[IBIS VER]   5.0
[File Name]   am13e230pn.ibs
[File Rev]   1.0
[Date]   February 08, 2026
[Source]   File originated at Texas Instruments
[Copyright]   (c) 2012, Texas Instruments Inc.
[Component]   am13e230pn
[Manufacturer] Texas Instruments
[Package]
| Variable   Typ   Min   Max
   R_pkg 2.94E-01 1.43E-01 3.97E-01
   L_pkg 6.08E-09 4.47E-09 7.53E-09
   C_pkg 1.84E-14 1.43E-14 3.70E-14
[Pin]   signal_name   model_name   R_pin   L_pin   C_pin
   1   VDD   NC 3.05E-01 6.58E-09 3.04E-14
   2   PB13   BCF3385DSWHYPBFZSD_87U 2.86E-01 6.29E-09 1.79E-14
   3   PB14   BCF3385DSHYPBFZSD_87U 2.74E-01 6.08E-09 1.74E-14
   4   PB15   BCF3385DSHYPBFZSD_87U 2.65E-01 5.90E-09 1.69E-14
   5 PC16_X1   BCF3385DSHYPBFZSD_87U 2.78E-01 5.95E-09 1.66E-14
   6 PC17_X2   BCF3385DSHYPBFZSD_87U 2.78E-01 5.86E-09 1.62E-14
   7   NRST   BQ0491FSSD_XRSN_87U 2.72E-01 5.71E-09 1.57E-14
   8   PB0   BCF3385DSHYPBFZSD_87U 2.65E-01 5.55E-09 1.53E-14
   9   PB1   BCF3385DSWHYPBFZSD_87U 2.61E-01 5.42E-09 1.48E-14
   10   PB2   BCF3385DSHYPBFZSD_87U 2.60E-01 5.32E-09 1.44E-14
   11   PB3   BCF3385DSHYPBFZSD_87U 2.60E-01 5.32E-09 1.44E-14
   12   PA0   BCF3385DSWHYPBFZSD_87U 2.59E-01 5.40E-09 1.48E-14
   13   PA1   BCF3385DSHYPBFZSD_87U 2.57E-01 5.47E-09 1.52E-14
   14   PA2   BCF3385DSWHYPBFZSD_87U 2.58E-01 5.56E-09 1.56E-14
   15   VSSA   NC 1.43E-01 4.47E-09 1.80E-14
   16   VDDA   NC 1.45E-01 4.57E-09 1.84E-14
   17   PA3   BCF3385DSHYPBFZSD_87U 2.71E-01 5.96E-09 1.70E-14
   18   PA4   BCF3385DSHYPBFZSD_87U 3.06E-01 6.41E-09 1.76E-14
   19   PA5   BCF3385DSHYPBFZSD_87U 3.26E-01 6.71E-09 1.82E-14
   20   PA6   BCF3385DSHYPBFZSD_87U 3.50E-01 7.04E-09 3.11E-14
   21   PA7   BCF3385DSHYPBFZSD_87U 3.54E-01 7.09E-09 3.12E-14
   22   PB4   BCF3385DSHYPBFZSD_87U 3.40E-01 6.85E-09 1.83E-14
   23   PB5   BCF3385DSWHYPBFZSD_87U 3.28E-01 6.64E-09 1.78E-14
   24   PA16   BCF3385DSHYPBFZSD_87U 3.19E-01 6.47E-09 1.73E-14
   25   PA17   BCF3385DSHYPBFZSD_87U 3.13E-01 6.31E-09 1.69E-14
   26   PA18   BCF3385DSHYPBFZSD_87U 3.09E-01 6.18E-09 1.64E-14
   27   VREFLO   NC 3.09E-01 6.09E-09 1.60E-14
   28   VREFHI   NC 3.09E-01 6.01E-09 1.56E-14
   29   VDDA   NC 3.14E-01 5.97E-09 1.52E-14
   30   PC7   BCF3385DSHYPBFZSD_87U 3.13E-01 5.87E-09 1.48E-14
   31   PC8   BCF3385DSHYPBFZSD_87U 3.10E-01 5.84E-09 1.48E-14
   32   PC9   BCF3385DSHYPBFZSD_87U 3.08E-01 5.91E-09 1.52E-14
   33   PC10   BCF3385DSHYPBFZSD_87U 3.09E-01 6.00E-09 1.56E-14
   34   PC11   BCF3385DSHYPBFZSD_87U 3.12E-01 6.12E-09 1.60E-14
   35   PC12   BCF3385DSHYPBFZSD_87U 3.17E-01 6.26E-09 1.65E-14
   36   PC13   BCF3385DSHYPBFZSD_87U 3.24E-01 6.43E-09 1.70E-14
   37   PC14   BCF3385DSHYPBFZSD_87U 3.34E-01 6.62E-09 1.75E-14
   38   PC15   BCF3385DSHYPBFZSD_87U 3.47E-01 6.84E-09 1.80E-14
   39   PA26   BCF3385DSHYPBFZSD_87U 3.62E-01 7.08E-09 1.85E-14
   40   VSS   NC 2.02E-01 5.52E-09 3.70E-14
   41   VDD   NC 3.75E-01 7.30E-09 3.15E-14
   42   PA27   BCF3385DSHYPBFZSD_87U 3.50E-01 6.95E-09 1.84E-14
   43   PA28   BCF3385DSHYPBFZSD_87U 3.38E-01 6.75E-09 1.79E-14
   44   PA29   BCF3385DSHYPBFZSD_87U 3.30E-01 6.57E-09 1.74E-14
   45   PA30   BCF3385DSHYPBFZSD_87U 3.24E-01 6.42E-09 1.69E-14
   46   PA31   BCF3385DSHYPBFZSD_87U 3.20E-01 6.29E-09 1.65E-14
   47   PB24   BCF3385DSHYPBFZSD_87U 3.18E-01 6.18E-09 1.61E-14
   48   PB25   BCF3385DSHYPBFZSD_87U 3.17E-01 6.09E-09 1.57E-14
   49   PB26   BCF3385DSHYPBFZSD_87U 3.18E-01 6.01E-09 1.53E-14
   50   VSS   NC 3.25E-01 5.99E-09 1.49E-14
   51   VDD   NC 3.25E-01 5.99E-09 1.49E-14
   52   PB6   BCF3385DSHYPBFZSD_87U 3.21E-01 6.04E-09 1.53E-14
   53   PB7   BCF3385DSHYPBFZSD_87U 3.24E-01 6.16E-09 1.57E-14
   54   PB8   BCF3385DSHYPBFZSD_87U 3.22E-01 6.22E-09 1.61E-14
   55   PB9   BCF3385DSHYPBFZSD_87U 3.26E-01 6.36E-09 1.66E-14
   56   PA8   BCF3385DSHYPBFZSD_87U 3.33E-01 6.52E-09 1.70E-14
   57   PA9   BCF3385DSHYPBFZSD_87U 3.43E-01 6.70E-09 1.75E-14
   58   PA10   BCF3385DSHYPBFZSD_87U 3.54E-01 6.91E-09 1.80E-14
   59   PA11   BCF3385DSHYPBFZSD_87U 3.52E-01 6.97E-09 1.84E-14
   60   PA12  BCPF335585DSHYPBFZSD_87U 3.67E-01 7.21E-09 3.13E-14
   61   VSS   NC 3.64E-01 7.19E-09 3.13E-14
   62   VDD   NC 1.80E-01 5.20E-09 2.07E-14
   63   PA13 BCF3385DSHYPBFZSD_TMS_87U 3.11E-01 6.47E-09 1.77E-14
   64   PA14 BCF3385DSHYPBFZSD_TMS_87U 2.63E-01 5.89E-09 1.69E-14
   65   PA15  BCPF335585DSHYPBFZSD_87U 2.55E-01 5.71E-09 1.64E-14
   66   PB10   BCF3385DSHYPBFZSD_87U 2.49E-01 5.57E-09 1.60E-14
   67   PB11   BCF3385DSHYPBFZSD_87U 2.47E-01 5.46E-09 1.56E-14
   68   PB12   BCF3385DSHYPBFZSD_87U 2.47E-01 5.37E-09 1.51E-14
   69   PB16   BCF3385DSHYPBFZSD_87U 2.48E-01 5.29E-09 1.47E-14
   70   PB17   BCF3385DSHYPBFZSD_87U 2.50E-01 5.23E-09 1.43E-14
   71   PB18  BCPF335585DSHYPBFZSD_87U 2.52E-01 5.24E-09 1.43E-14
   72   PA19  BCPF335585DSHYPBFZSD_87U 2.49E-01 5.30E-09 1.47E-14
   73   PA20   BCF3385DSHYPBFZSD_87U 2.51E-01 5.40E-09 1.52E-14
   74   PA21   BCF3385DSHYPBFZSD_87U 2.52E-01 5.50E-09 1.56E-14
   75   PA22   BCF3385DSHYPBFZSD_87U 2.57E-01 5.65E-09 1.60E-14
   76   PA23   BCF3385DSHYPBFZSD_87U 2.66E-01 5.82E-09 1.65E-14
   77   PA24   BCF3385DSHYPBFZSD_87U 2.74E-01 5.99E-09 1.70E-14
   78   PA25   BCF3385DSHYPBFZSD_87U 2.87E-01 6.22E-09 1.75E-14
   79   VSS   NC 1.64E-01 5.04E-09 2.02E-14
   80   VDD   NC 3.01E-01 6.54E-09 3.04E-14
| End of package information
|   Component BCF3385DSHYPBFZSD_87U
[Component] BCF3385DSHYPBFZSD_87U
[Manufacturer] Texas Instruments
[Package]
| variable   typ   min   max
R_pkg   0.0   0.0   0.0
L_pkg   0.0H   0.0H   0.0H
C_pkg   0.0F   0.0F   0.0F
[Pin]  signal_name   model_name   R_pin   L_pin   C_pin
PAD   PAD   BCF3385DSHYPBFZSD_87U
VDDS   VDDS   Power
VSS   VSS   Gnd
A   A   NC
GZ   GZ   NC
[Model Selector] BCF3385DSHYPBFZSD_87U
BCF3385DSHYPBFZSD_87U_PUPDOFF PI=1 PSEL=1
BCF3385DSHYPBFZSD_87U_PDON PI=0 PSEL=0
BCF3385DSHYPBFZSD_87U_PUON PI=0 PSEL=1
|   Component BCF3385DSHYPBFZSD_TMS_87U
[Component] BCF3385DSHYPBFZSD_TMS_87U
[Manufacturer] Texas Instruments
[Package]
| variable   typ   min   max
R_pkg   0.0   0.0   0.0
L_pkg   0.0H   0.0H   0.0H
C_pkg   0.0F   0.0F   0.0F
[Pin]  signal_name   model_name   R_pin   L_pin   C_pin
PAD   PAD   BCF3385DSHYPBFZSD_TMS_87U
VDDS   VDDS   Power
VSS   VSS   Gnd
A   A   NC
GZ   GZ   NC
[Model Selector] BCF3385DSHYPBFZSD_TMS_87U
BCF3385DSHYPBFZSD_TMS_87U_PUPDOFF PI=1 PSEL=1
BCF3385DSHYPBFZSD_TMS_87U_PDON PI=0 PSEL=0
BCF3385DSHYPBFZSD_TMS_87U_PUON PI=0 PSEL=1
|   Component BCF3385DSWHYPBFZSD_87U
[Component] BCF3385DSWHYPBFZSD_87U
[Manufacturer] Texas Instruments
[Package]
| variable   typ   min   max
R_pkg   0.0   0.0   0.0
L_pkg   0.0H   0.0H   0.0H
C_pkg   0.0F   0.0F   0.0F
[Pin]  signal_name   model_name   R_pin   L_pin   C_pin
PAD   PAD   BCF3385DSWHYPBFZSD_87U
VDDS   VDDS   Power
VSS   VSS   Gnd
A   A   NC
GZ   GZ   NC
[Model Selector] BCF3385DSWHYPBFZSD_87U
BCF3385DSWHYPBFZSD_87U_PUPDOFF PI=1 PSEL=1
BCF3385DSWHYPBFZSD_87U_PDON PI=0 PSEL=0
BCF3385DSWHYPBFZSD_87U_PUON PI=0 PSEL=1
|   Component BCPF335585DSHYPBFZSD_87U
[Component] BCPF335585DSHYPBFZSD_87U
[Manufacturer] Texas Instruments
[Package]
| variable   typ   min   max
R_pkg   0.0   0.0   0.0
L_pkg   0.0H   0.0H   0.0H
C_pkg   0.0F   0.0F   0.0F
[Pin]  signal_name   model_name   R_pin   L_pin   C_pin
PAD   PAD   BCPF335585DSHYPBFZSD_87U
VDDS   VDDS   Power
VSS   VSS   Gnd
A   A   NC
GZ   GZ   NC
[Model Selector] BCPF335585DSHYPBFZSD_87U
BCPF335585DSHYPBFZSD_87U_PUPDOFF_D0 DS=0
BCPF335585DSHYPBFZSD_87U_PUPDOFF_D1 DS=1
BCPF335585DSHYPBFZSD_87U_PDON PI=0 PSEL=0
BCPF335585DSHYPBFZSD_87U_PUON PI=0 PSEL=1
|   Component BQ0491FSSD_XRSN_87U
[Component] BQ0491FSSD_XRSN_87U
[Manufacturer] Texas Instruments
[Package]
| variable   typ   min   max
R_pkg   0.0   0.0   0.0
L_pkg   0.0H   0.0H   0.0H
C_pkg   0.0F   0.0F   0.0F
[Pin]  signal_name   model_name   R_pin   L_pin   C_pin
PAD   PAD   BQ0491FSSD_XRSN_87U
VDDS   VDDS   Power
VSS   VSS   Gnd
A   A   NC
[Model Selector] BQ0491FSSD_XRSN_87U
BQ0491FSSD_XRSN_87U_PUPDOFF PI=1
BQ0491FSSD_XRSN_87U_PUPDON PI=0
| Models and submodels in the file (15): BCF3385DSHYPBFZSD_87U_PUPDOFF (I/O), BCF3385DSHYPBFZSD_87U_PDON (Input), BCF3385DSHYPBFZSD_87U_PUON (Input), BCF3385DSHYPBFZSD_TMS_87U_PUPDOFF (I/O), BCF3385DSHYPBFZSD_TMS_87U_PDON (Input), BCF3385DSHYPBFZSD_TMS_87U_PUON (Input), BCF3385DSWHYPBFZSD_87U_PUPDOFF (I/O), BCF3385DSWHYPBFZSD_87U_PDON (Input), BCF3385DSWHYPBFZSD_87U_PUON (Input), BCPF335585DSHYPBFZSD_87U_PUPDOFF_D0 (I/O), BCPF335585DSHYPBFZSD_87U_PUPDOFF_D1 (I/O), BCPF335585DSHYPBFZSD_87U_PDON (Input), BCPF335585DSHYPBFZSD_87U_PUON (Input), BQ0491FSSD_XRSN_87U_PUPDOFF (Input), BQ0491FSSD_XRSN_87U_PUPDON (Input)
